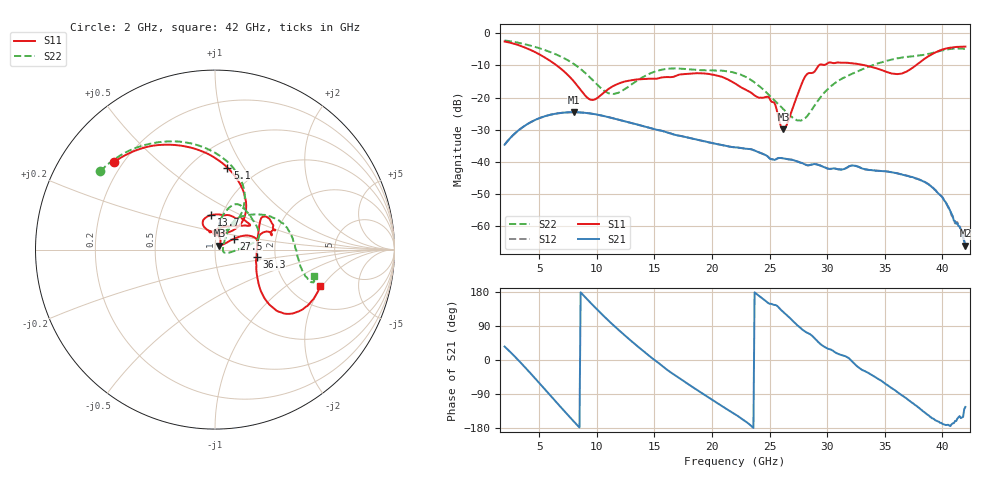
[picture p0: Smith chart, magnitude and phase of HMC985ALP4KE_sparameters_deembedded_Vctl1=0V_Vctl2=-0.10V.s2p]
!s2p File: Measurements: S11, S21, S12, S22
# GHz S dB R 50.0
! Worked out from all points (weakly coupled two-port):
!   401 points, 2 GHz to 42 GHz, reference 50 ohm
!   highest |S21| = -24.50 dB at 8 GHz (marker M1); lowest = -66.0 dB at 42 GHz (marker M2)
!   lowest |S11| = -29.8 dB at 26.2 GHz (marker M3), VSWR 1.07, Z = 52.5 + j2.21 ohm
!   |S11| at or under -10 dB: 6.527 GHz to 29.27 GHz (22.75 GHz wide, 127 % of centre); 33.34 GHz to 37.69 GHz (4.35 GHz wide, 12.2 % of centre)
!   |S22| runs from -27.1 to -2.2 dB; largest |S21 - S12| = 0.00014
!   S11 on the Smith chart (normalised r, x): 2 GHz: 0.17, +0.36; 5.1 GHz: 0.73, +0.85; 13.7 GHz: 0.89, +0.35; 27.5 GHz: 1.22, +0.15; 36.3 GHz: 1.59, -0.14; 42 GHz: 2.90, -1.92
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2  -2.55 139.3  -34.62 35.4  -34.62 35.4  -2.23 145.6
3.5  -4.07 111.4  -29.34 -10.4  -29.34 -10.4  -3.18 121.9
5.1  -6.71 81.4  -26.24 -63.8  -26.25 -63.8  -4.74 97.5
8  -14.90 44.8  -24.50 -162.0  -24.51 -162.0  -9.50 60.3
8.7  -18.07 51.5  -24.61 175.2  -24.62 175.1  -11.39 55.0
9.7  -20.69 87.3  -25.04 143.4  -25.04 143.4  -14.74 52.7
11.2  -16.88 115.8  -26.20 98.6  -26.20 98.6  -18.77 67.5
13.7  -14.29 96.7  -28.52 32.1  -28.52 32.1  -14.26 77.3
15.4  -13.94 73.0  -30.08 -8.7  -30.09 -8.8  -11.51 68.3
19.4  -12.51 34.7  -33.61 -92.8  -33.60 -92.9  -11.49 34.3
22  -15.56 52.2  -35.43 -143.0  -35.43 -142.9  -12.27 13.3
25  -20.24 97.6  -38.82 148.6  -38.84 148.5  -19.34 -4.0
26.2  -29.83 40.7  -38.87 126.4  -38.85 126.3  -23.59 -16.5
27.5  -18.43 29.5  -39.92 89.5  -39.94 89.6  -27.06 -3.8
28.1  -13.37 20.6  -40.78 74.7  -40.72 74.7  -26.35 20.1
28.7  -12.32 12.7  -40.76 63.7  -40.75 63.7  -23.57 39.0
31  -9.09 23.4  -42.28 15.7  -42.21 15.8  -14.69 56.9
33.3  -9.96 34.5  -42.26 -29.7  -42.26 -29.8  -10.86 42.9
35.4  -12.27 12.5  -43.08 -69.9  -43.02 -69.9  -8.35 26.1
36.3  -12.57 -10.1  -43.71 -89.4  -43.71 -89.3  -7.67 18.2
39.9  -5.18 -40.5  -50.57 -165.8  -50.58 -166.2  -5.41 -17.0
42  -4.14 -19.0  -65.97 -124.0  -66.11 -121.8  -4.88 -14.8
